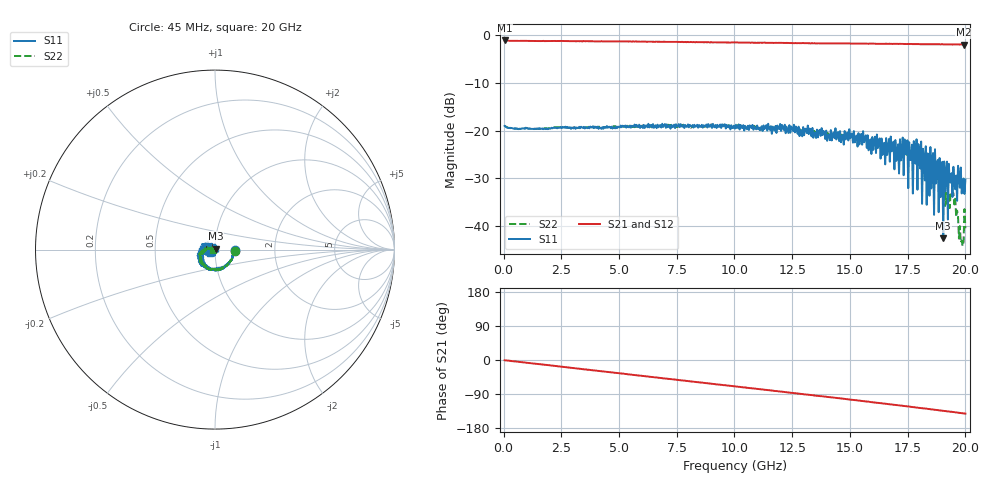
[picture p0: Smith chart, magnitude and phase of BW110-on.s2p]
!  2-Port S-parameters saved by WinCal
! VAR MeasName=S-Parameters (CALIBRATED_DATA) read from VNA (E8364A)
! VAR MeasDate=10/9/2010 2:19:22 PM
! VAR NAME=15(25)on
! VAR FILENAME=15(25)on.s2p
! VAR DATE=10/9/2010 2:19:23 PM
! VAR PHYS_PORTS=1,2
# Hz S RI R 50
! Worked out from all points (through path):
!   501 points, 45 MHz to 20 GHz, reference 50 ohm
!   highest |S21| = -1.14 dB at 45 MHz (marker M1); lowest = -2.0 dB at 19.92 GHz (marker M2)
!   group delay of S21, straight-line fit = 19.4 ps
!   lowest |S11| = -42.6 dB at 19.04 GHz (marker M3), VSWR 1.01, Z = 50.5 + j0.589 ohm
!   |S11| at or under -10 dB: start of sweep to end of sweep
!   |S22| runs from -44.2 to -18.7 dB; largest |S21 - S12| = 0.006
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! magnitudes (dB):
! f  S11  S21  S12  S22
! 45 MHz  -19.0  -1.1  -1.1  -19.0
! 3.397 GHz  -19.4  -1.3  -1.3  -19.4
! 6.71 GHz  -19.3  -1.4  -1.4  -19.1
! 10.02 GHz  -19.6  -1.6  -1.6  -19.2
! 13.37 GHz  -19.5  -1.7  -1.7  -19.9
! 15.09 GHz  -20.6  -1.8  -1.8  -20.9
! 16.69 GHz  -21.8  -1.8  -1.8  -24.1
! 17.05 GHz  -24.5  -1.8  -1.8  -24.0
! 17.33 GHz  -29.4  -1.9  -1.9  -25.8
! 17.57 GHz  -22.4  -1.9  -1.9  -24.7
! 17.92 GHz  -32.4  -1.9  -1.9  -27.1
! 18.16 GHz  -23.8  -1.9  -1.9  -26.4
! 18.36 GHz  -24.8  -1.9  -1.9  -27.7
! 18.52 GHz  -32.1  -1.9  -1.9  -30.5
! 18.84 GHz  -37.1  -1.9  -1.9  -29.7
! 19.04 GHz  -42.6  -2.0  -2.0  -33.4
! 19.2 GHz  -26.5  -2.0  -2.0  -35.2
! 19.48 GHz  -27.6  -2.0  -2.0  -33.1
! 19.76 GHz  -32.0  -2.0  -2.0  -40.0
! 19.8 GHz  -27.7  -2.0  -2.0  -43.4
! 19.92 GHz  -30.0  -2.0  -2.0  -43.4
! 20 GHz  -30.3  -2.0  -2.0  -40.5
